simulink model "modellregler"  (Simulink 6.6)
settings: Solver=ode1  StartTime=0.0  StopTime=10000  FixedStep=0.01  RelTol=1e-3
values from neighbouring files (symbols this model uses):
  a = 2*(Va/ha)    (= 0.346988908589)    [regler.m]
  A = Vt/ht    [regler.m]
  g = 9.81    [regler.m]
  Kq = ausgang_ein/(zufall(i)+10)    [regler.m]
  stoergroesse = ausgang_ein/8    (= 5.625)    [regler.m]
libraries: simulink_extras x1

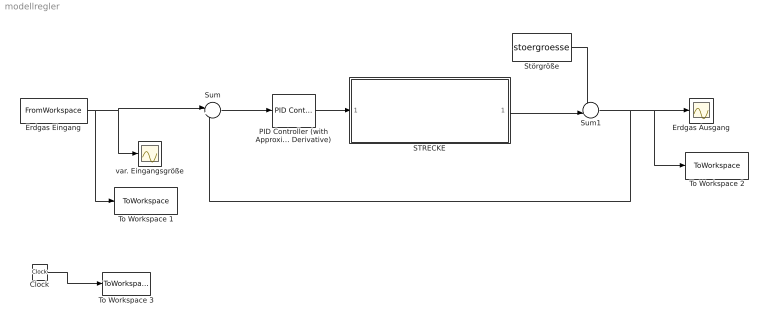
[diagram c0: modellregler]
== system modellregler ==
  Clock : Clock
  Erdgas Ausgang : Scope
  Erdgas Eingang : FromWorkspace  VariableName=eingang_ein  SampleTime=0
  PID Controller (with Approximate Derivative) : simulink_extras/Additional Linear/PID Controller (with Approximate Derivative)  SystemSampleTime=-1  P=10  I=10  D=240  N=10
  STRECKE : Subsystem
  Störgröße : Constant  Value=stoergroesse
  Sum : Sum  Inputs=|+-
  Sum1 : Sum  Inputs=-+|
  To Workspace 1 : ToWorkspace  VariableName=eingang_aus  SampleTime=-1  SaveFormat=Array
  To Workspace 2 : ToWorkspace  VariableName=ausgang_aus  SampleTime=-1  SaveFormat=Array
  To Workspace 3 : ToWorkspace  VariableName=zeit  SampleTime=-1  SaveFormat=Array
  var. Eingangsgröße : Scope
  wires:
  Clock/1 -> To Workspace 3/1
  Erdgas Eingang/1 -> To Workspace 1/1, var. Eingangsgröße/1, Sum/1
  Sum/1 -> PID Controller (with Approximate Derivative)/1
  PID Controller (with Approximate Derivative)/1 -> STRECKE/1(eingang)
  STRECKE/1(ausgang) -> Sum1/2
  Sum1/1 -> Erdgas Ausgang/1, To Workspace 2/1, Sum/2
  Störgröße/1 -> Sum1/1

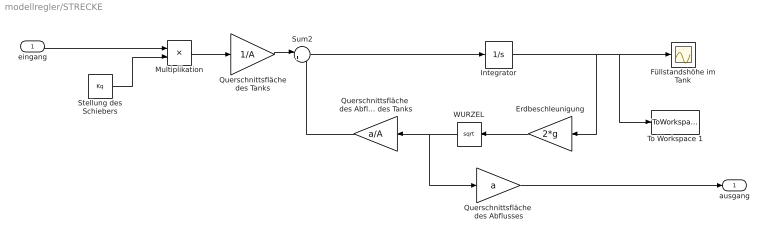
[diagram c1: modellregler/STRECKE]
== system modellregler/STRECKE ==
  eingang : Inport
  Erdbeschleunigung : Gain  Orientation=left  Gain=2*g
  Füllstandshöhe im Tank : Scope
  Integrator : Integrator
  Multiplikation : Product
  Querschnittsfläche  des Abflusses : Gain  Gain=a
  Querschnittsfläche  des Abflusses / Querschnittsfläche des Tanks : Gain  Orientation=left  Gain=a/A
  Querschnittsfläche des Tanks : Gain  Gain=1/A
  Stellung des Schiebers : Constant  Value=Kq
  Sum2 : Sum  Inputs=|+-
  To Workspace 1 : ToWorkspace  VariableName=fuellhoehe  SampleTime=-1  SaveFormat=Array
  WURZEL : Math  Orientation=left  Operator=sqrt
  ausgang : Outport
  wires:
  eingang/1 -> Multiplikation/1
  Stellung des Schiebers/1 -> Multiplikation/2
  Sum2/1 -> Integrator/1
  Integrator/1 -> Erdbeschleunigung/1, Füllstandshöhe im Tank/1, To Workspace 1/1
  Erdbeschleunigung/1 -> WURZEL/1
  WURZEL/1 -> Querschnittsfläche  des Abflusses / Querschnittsfläche des Tanks/1, Querschnittsfläche  des Abflusses/1
  Querschnittsfläche des Tanks/1 -> Sum2/1
  Querschnittsfläche  des Abflusses / Querschnittsfläche des Tanks/1 -> Sum2/2
  Querschnittsfläche  des Abflusses/1 -> ausgang/1
  Multiplikation/1 -> Querschnittsfläche des Tanks/1
